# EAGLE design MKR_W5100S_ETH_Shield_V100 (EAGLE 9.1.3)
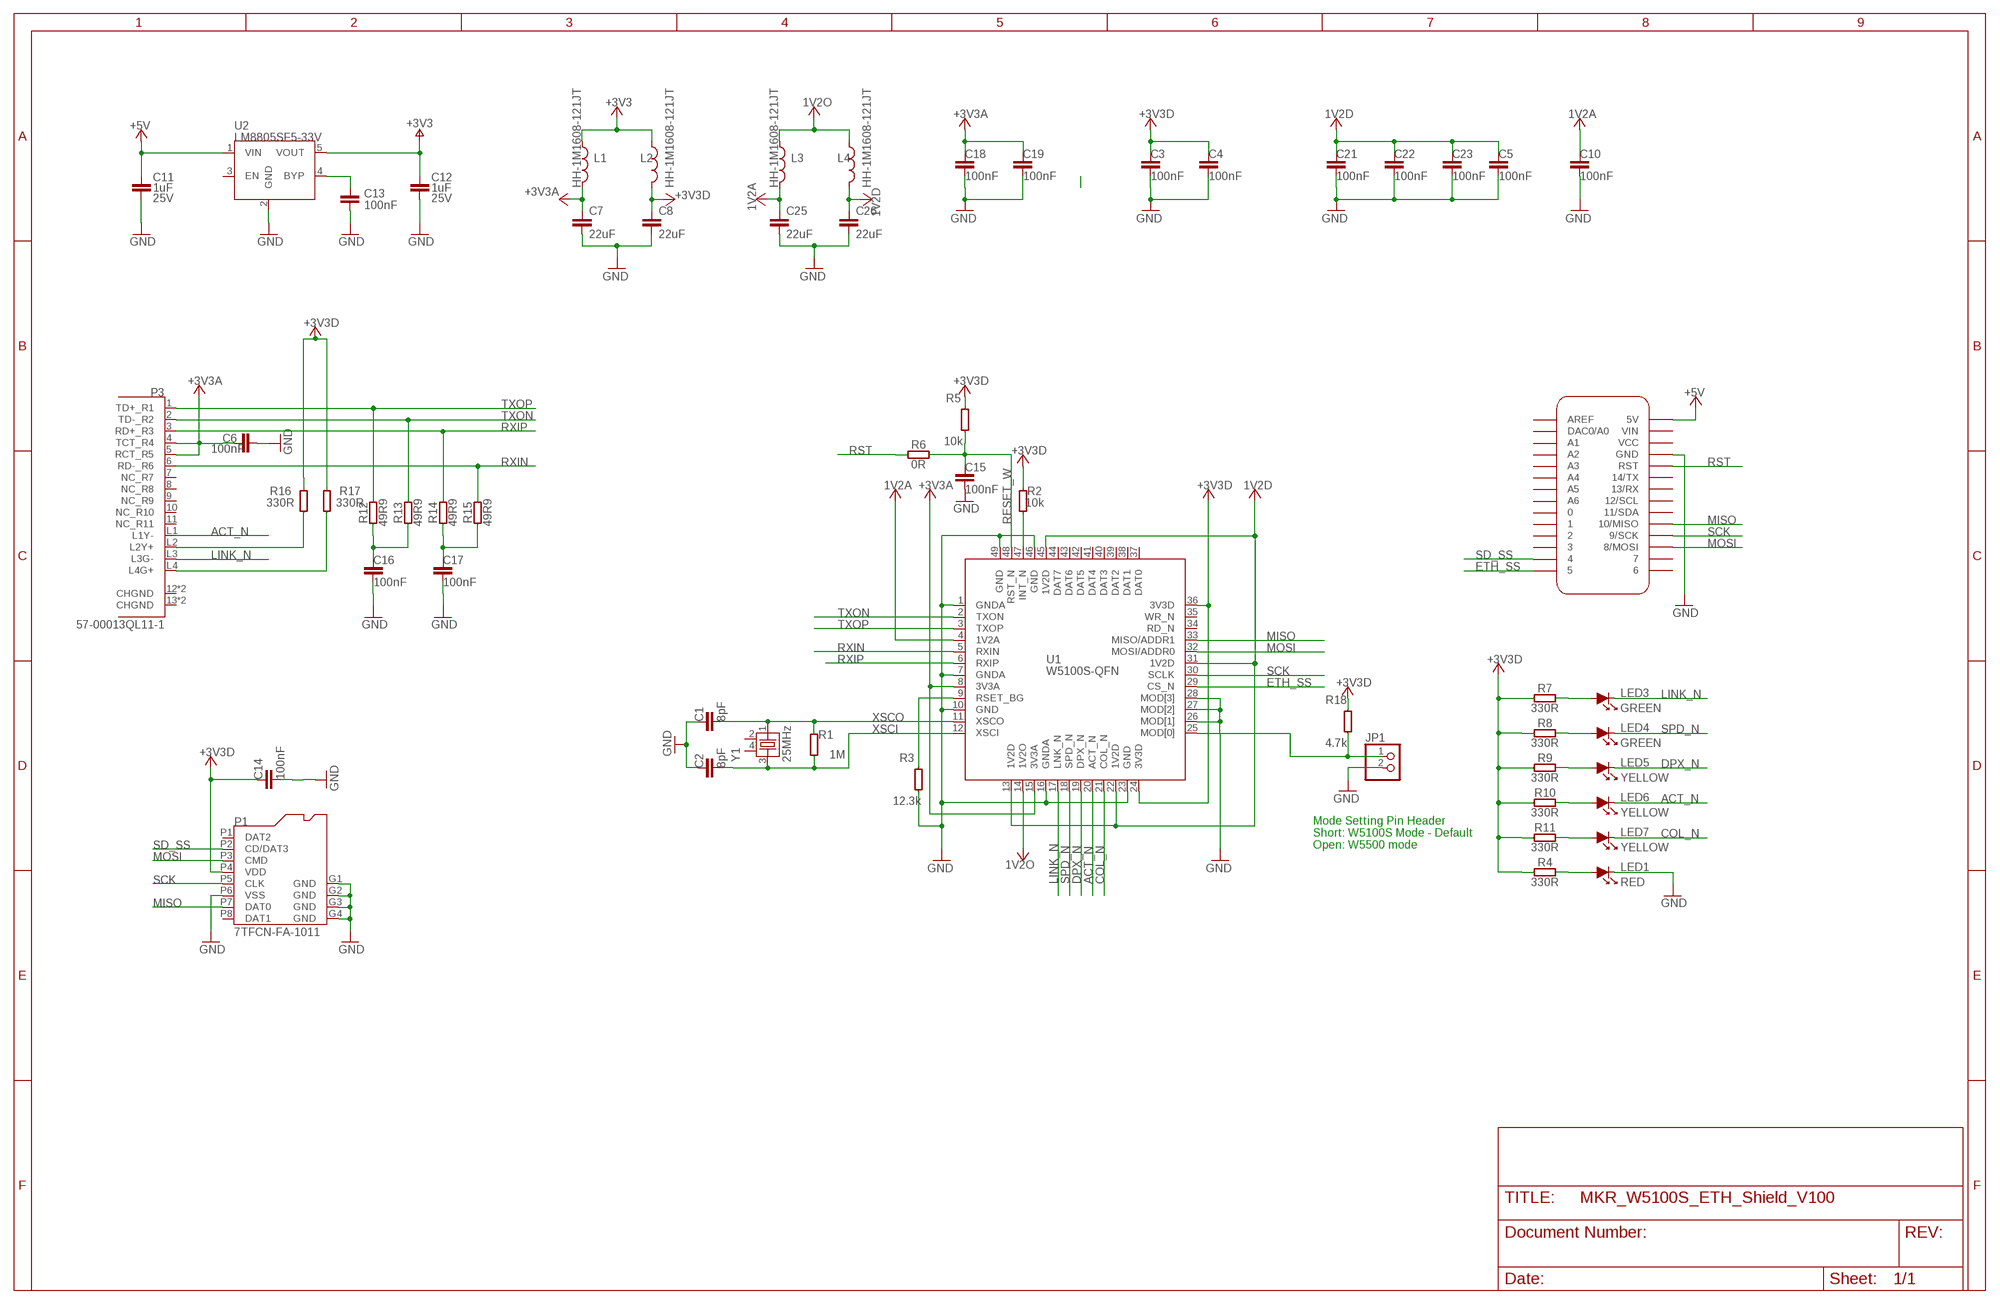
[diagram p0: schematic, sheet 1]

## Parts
C1  8pF  C-1UF-0402  [0402-1005X55N]
C2  8pF  C-1UF-0402  [0402-1005X55N]
C3  100nF  C-1UF-0402  [0402-1005X55N]
C4  100nF  C-1UF-0402  [0402-1005X55N]
C5  100nF  C-1UF-0402  [0402-1005X55N]
C6  100nF  C-1UF-0402  [0402-1005X55N]
C7  22uF  C-22U-0805  [0805-R2013X50N]
C8  22uF  C-22U-0805  [0805-R2013X50N]
C10  100nF  C-1UF-0402  [0402-1005X55N]
C11  1uF  C-1UF-0402  [0402-1005X55N]
C12  1uF  C-1UF-0402  [0402-1005X55N]
C13  100nF  C-100NF-0402  [0402-1005X55N]
C14  100nF  C-1UF-0402  [0402-1005X55N]
C15  100nF  C-1UF-0402  [0402-1005X55N]
C16  100nF  C-1UF-0402  [0402-1005X55N]
C17  100nF  C-1UF-0402  [0402-1005X55N]
C18  100nF  C-1UF-0402  [0402-1005X55N]
C19  100nF  C-1UF-0402  [0402-1005X55N]
C21  100nF  C-1UF-0402  [0402-1005X55N]
C22  100nF  C-1UF-0402  [0402-1005X55N]
C23  100nF  C-1UF-0402  [0402-1005X55N]
C25  22uF  C-22U-0805  [0805-R2013X50N]
C26  22uF  C-22U-0805  [0805-R2013X50N]
JP1  PINHD-1X2  [1X02]
L1  HH-1M1608-121JT  BLM18PG471SN1D  [0603-1608X90N]
L2  HH-1M1608-121JT  BLM18PG471SN1D  [0603-1608X90N]
L3  HH-1M1608-121JT  BLM18PG471SN1D  [0603-1608X90N]
L4  HH-1M1608-121JT  BLM18PG471SN1D  [0603-1608X90N]
LED1  RED  LED-1608  [LED-1608]
LED3  GREEN  LED-1608  [LED-1608]
LED4  GREEN  LED-1608  [LED-1608]
LED5  YELLOW  LED-1608  [LED-1608]
LED6  YELLOW  LED-1608  [LED-1608]
LED7  YELLOW  LED-1608  [LED-1608]
MKR1  DNP  ARDUINO-UTILITY_MKRBOARDNO-OUTLINE  [ARDUINO-UTILITY_MKRBOARD-NOOUTLINE]
P1  7TFCN-FA-1011  [7TFCN-FA-1011]
P3  57-00013QL11-1  [57-00013QL11-1]
R1  1M  R-330R-0402  [0402-1005X55N]
R2  10k  R-330R-0402  [0402-1005X55N]
R3  12.3k  R-330R-0402  [0402-1005X55N]
R4  330R  R-330R-0402  [0402-1005X55N]
R5  10k  R-330R-0402  [0402-1005X55N]
R6  0R  R-330R-0402  [0402-1005X55N]
R7  330R  R-330R-0402  [0402-1005X55N]
R8  330R  R-330R-0402  [0402-1005X55N]
R9  330R  R-330R-0402  [0402-1005X55N]
R10  330R  R-330R-0402  [0402-1005X55N]
R11  330R  R-330R-0402  [0402-1005X55N]
R12  49R9  R-330R-0402  [0402-1005X55N]
R13  49R9  R-330R-0402  [0402-1005X55N]
R14  49R9  R-330R-0402  [0402-1005X55N]
R15  49R9  R-330R-0402  [0402-1005X55N]
R16  330R  R-330R-0402  [0402-1005X55N]
R17  330R  R-330R-0402  [0402-1005X55N]
R18  4.7k  R-330R-0402  [0402-1005X55N]
U1  W5100S-QFN  [W5100S-QFN]
U2  LM8805SF5-33V  [SOT23-5L]
Y1  25MHz  XTAL3225  [XTAL3225]

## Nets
1V2A: C10.1 C25.1 L3.2 U1.4(1V2A)
1V2D: C5.1 C21.1 C22.1 C23.1 C26.1 L4.2 U1.13(1V2D) U1.22(1V2D) U1.31(1V2D) U1.45(1V2D)
1V2O: L3.1 L4.1 U1.14(1V2O)
+3V3 [power]: C12.1 L1.1 L2.1 U2.5(VOUT)
+3V3A [power]: C6.1 C7.1 C18.1 C19.1 L1.2 P3.4(TCT_R4) P3.5(RCT_R5) U1.8(3V3A) U1.15(3V3A)
+3V3D: C3.1 C4.1 C8.1 C14.1 L2.2 P1.P4(VDD) R2.1 R4.2 R5.2 R7.2 R8.2 R9.2 R10.2 R11.2 R16.1 R17.1 R18.2 U1.24(3V3D) U1.36(3V3D)
+5V: C11.1 MKR1.5V U2.1(VIN)
ACT_N: LED6.K P3.L1(L1Y-) U1.20(ACT_N)
COL_N: LED7.K U1.21(COL_N)
DPX_N: LED5.K U1.19(DPX_N)
ETH_SS: MKR1.5 U1.29(CS_N)
GND [gnd]: C1.1 C2.1 C3.2 C4.2 C5.2 C6.2 C7.2 C8.2 C10.2 C11.2 C12.2 C13.2 C14.2 C15.2 C16.2 C17.2 C18.2 C19.2 C21.2 C22.2 C23.2 C25.2 C26.2 JP1.2 LED1.K MKR1.GND P1.G1(GND) P1.G2(GND) P1.G3(GND) P1.G4(GND) P1.P6(VSS) R3.1 U1.1(GNDA) U1.7(GNDA) U1.10(GND) U1.16(GNDA) U1.23(GND) U1.26(MOD[1]) U1.27(MOD[2]) U1.28(MOD[3]) U1.46(GND) U1.49(GND) U2.2(GND)
LINK_N: LED3.K P3.L3(L3G-) U1.17(LNK_N)
MISO: MKR1.10(10/MISO) P1.P7(DAT0) U1.33(MISO/ADDR1)
MOSI: MKR1.8(8/MOSI) P1.P3(CMD) U1.32(MOSI/ADDR0)
N$1: LED3.A R7.1
N$2: P3.L2(L2Y+) R16.2
N$3: LED1.A R4.1
N$4: LED4.A R8.1
N$5: LED5.A R9.1
N$6: LED6.A R10.1
N$7: LED7.A R11.1
N$8: P3.L4(L4G+) R17.2
N$9: JP1.1 R18.1 U1.25(MOD[0])
N$11: C13.1 U2.4(BYP)
N$12: C16.1 R12.2 R13.2
N$15: C17.1 R14.2 R15.2
N$16: R2.2 U1.47(INT_N)
N$20: R3.2 U1.9(RSET_BG)
RESET_W: C15.1 R5.1 R6.1 U1.48(RST_N)
RST: MKR1.RST R6.2
RXIN: P3.6(RD-_R6) R15.1 U1.5(RXIN)
RXIP: P3.3(RD+_R3) R14.1 U1.6(RXIP)
SCK: MKR1.9(9/SCK) P1.P5(CLK) U1.30(SCLK)
SD_SS: MKR1.4 P1.P2(CD/DAT3)
SPD_N: LED4.K U1.18(SPD_N)
TXON: P3.2(TD-_R2) R13.1 U1.2(TXON)
TXOP: P3.1(TD+_R1) R12.1 U1.3(TXOP)
XSCI: C2.2 R1.1 U1.12(XSCI) Y1.3
XSCO: C1.2 R1.2 U1.11(XSCO) Y1.1
Unconnected: MKR1.0 MKR1.1 MKR1.2 MKR1.3 MKR1.6 MKR1.7 MKR1.11(11/SDA) MKR1.12(12/SCL) MKR1.13(13/RX) MKR1.14(14/TX) MKR1.A0(DAC0/A0) MKR1.A1 MKR1.A2 MKR1.A3 MKR1.A4 MKR1.A5 MKR1.A6 MKR1.AREF MKR1.VCC MKR1.VIN P1.P1(DAT2) P1.P8(DAT1) P3.7(NC_R7) P3.8(NC_R8) P3.9(NC_R9) P3.10(NC_R10) P3.11(NC_R11) P3.12(CHGND) P3.13(CHGND) P3.P$3(CHGND) P3.P$4(CHGND) U1.34(RD_N) U1.35(WR_N) U1.37(DAT0) U1.38(DAT1) U1.39(DAT2) U1.40(DAT3) U1.41(DAT4) U1.42(DAT5) U1.43(DAT6) U1.44(DAT7) U2.3(EN) Y1.2 Y1.4

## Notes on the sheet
- Mode Setting Pin Header
  Short: W5100S Mode - Default
  Open: W5500 mode

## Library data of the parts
C1-C6 C10-C12 C14-C19 C21-C23 = MK1_Zero:C: Capacitor; DESCR: CAP CER 1UF 25V 10% X5R 0402; MF: Murata; MPN: GRM155R61E105KA12D; VOLTAGE: 25V
C7 C8 C25 C26 = Arduino-rcl:C: SMD Capacitor; CODE-ARDUINO: 2233; DATASHEET: https://media.digikey.com/pdf/Data%20Sheets/Samsung%20PDFs/CL21A226MQCLQNC_character.pdf; DISTRIBUTOR-LINK: https://www.digikey.com/product-detail/en/samsung-electro-mechanics-america-inc/CL21A226MQCLQNC/1276-2412-1-ND/3890498; DISTRIBUTOR-PN: 1276-2412-1-ND; MANUFACTURER: Samsung; MANUFACTURER-PN: CL21A226MQCLQNC; VALUE: 22u
C13 = MK1_Zero:C: Capacitor; DESCR: CAP CER 0.1UF 50V 10% X5R 0402; MF: TDK; MPN: C1005X5R1H104K050BB
JP1 = PinHeader:PINHD-1X2: PIN HEADER
L1-L4 = MK1_Zero:BLM18PG471SN1D: FERRITE CHIP 470 OHM 1000MA 0603
LED1 LED3-LED7 = DIODE:LED-1608
MKR1 = MKRETHShieldV2.0:ARDUINO-UTILITY_MKRBOARD: MKR board footprint; DATASHEET: DNP; DISTRIBUTOR-LINK: DNP; DISTRIBUTOR-PN: DNP; MANUFACTURER: DNP; MANUFACTURER-PN: DNP
P1 = Connector:7TFCN-FA-1011
P3 = WIZnet:57-00013QL11-1
R1-R18 = MK1_Zero:R: Resistor; DESCR: RES 330 OHM 1/16W 1% 0402 SMD; MF: Yageo; MPN: RC0402FR-07330RL
U1 = WIZnet:W5100S-QFN
U2 = RECULATOR:LM8805SF5-33V
Y1 = X-TAL:XTAL3225

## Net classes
1 power: width 0.254 mm, drill 0.3 mm, clearance 0.127 mm
2 gnd: width 0.254 mm, drill 0.3 mm, clearance 0.127 mm

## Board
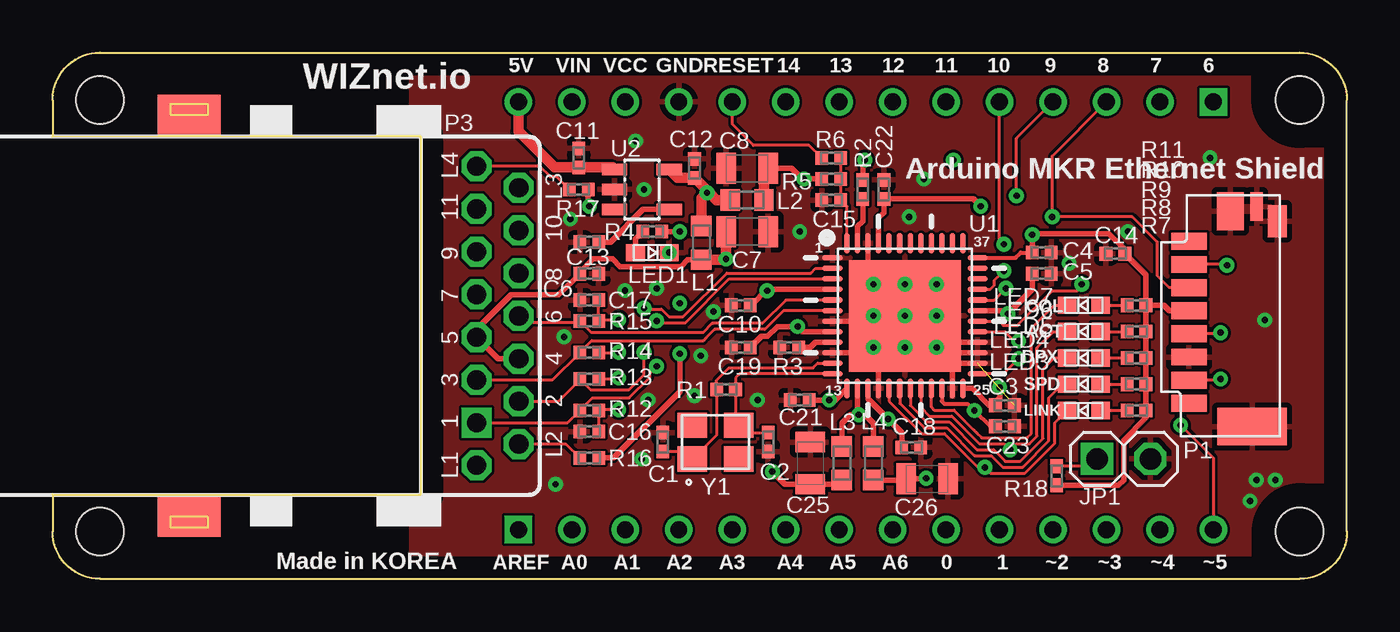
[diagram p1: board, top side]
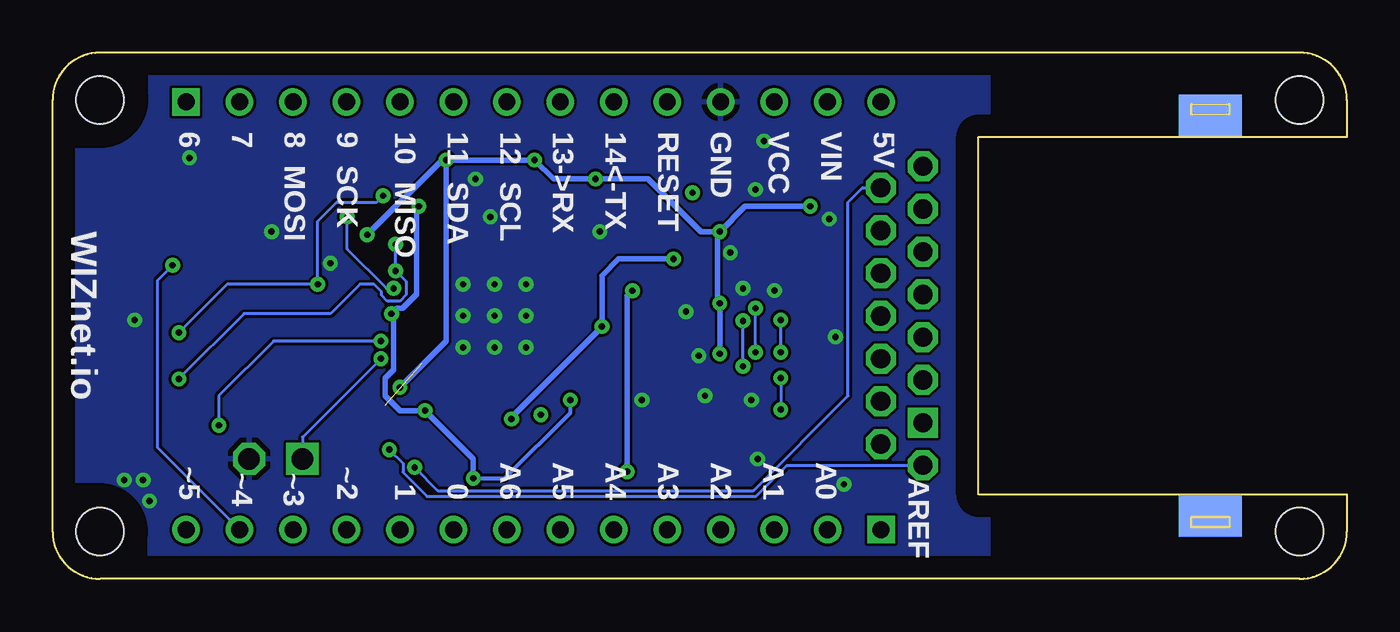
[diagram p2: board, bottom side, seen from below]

Size 61.5 x 25 mm. Coordinates in mm from the lower left corner, seen from the top.
Outline: 2.25,0 59.25,0 arc90 61.5,2.25 61.5,22.75 arc90 59.25,25 2.25,25 arc90 0,22.75 0,21 17.5,21 17.5,4 0,4 0,2.25 arc90 2.25,0
Copper layers (1*16): Top 0.035mm / dielectric 1.5mm / Bottom 0.035mm
Design rules "default *": minimum track width 6mil, minimum drill 0.3mm, track to track 5mil, track to pad 5mil, pad to pad 5mil, via to via 5mil, smd to smd 5mil, copper to edge 40mil, drill to drill 6mil, minimum pad ring 10mil, minimum via ring 8mil, stop-mask expansion 4mil, vias tented up to drill 15mil, thermal gap 10mil
Holes 2.25 mm at 2.25,2.25 2.25,22.75 59.25,2.25 59.25,22.75
tRestrict: area 57,20.5 to 61.5,25; area 57,0 to 61.5,4.5; 4 lines
bRestrict: area 57,20.5 to 61.5,25; area 57,0 to 61.5,4.5; 4 lines

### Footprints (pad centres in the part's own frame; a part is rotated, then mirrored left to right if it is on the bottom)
0402-1005X55N = smd 0.62 x 0.62: 1 -0.45,0; 2 0.45,0
0805-R2013X50N = smd 0.95 x 1.45: 1 -1,0; 2 1,0
1X02 = drill 1.016 square: 1 -1.27,0 | drill 1.016 octagon: 2 1.27,0
0603-1608X90N = smd 0.95 x 1: 1 -0.8,0; 2 0.8,0
LED-1608 = smd 0.89 x 0.82: A -0.8,0; K 0.8,0
ARDUINO-UTILITY_MKRBOARD-NOOUTLINE = drill 0.8: 0 42.455,2.34; 1 44.995,2.34; 2 47.535,2.34; 3 50.075,2.34; 4 52.615,2.34; 5 55.155,2.34; 5V 22.135,22.66; 7 52.615,22.66; 8 50.075,22.66; 9 47.535,22.66; 10 44.995,22.66; 11 42.455,22.66; 12 39.915,22.66; 13 37.375,22.66; 14 34.835,22.66; A0 24.675,2.34; A1 27.215,2.34; A2 29.755,2.34; A3 32.295,2.34; A4 34.835,2.34; A5 37.375,2.34; A6 39.915,2.34; GND 29.755,22.66; RST 32.295,22.66; VCC 27.215,22.66; VIN 24.675,22.66 | drill 0.8 square: 6 55.155,22.66; AREF 22.135,2.34
7TFCN-FA-1011 = smd 1.8 x 3.3: G1 -5.26,0 | smd 1.8 x 1.3: G2 4.97,1.04 | smd 1.36 x 0.6: G3 5.19,-0.21 | smd 1.5 x 0.9: G4 4.49,-1.2 | smd 0.8 x 1.7: P1 3.54,3; P2 2.44,3; P3 1.34,3; P4 0.24,3; P5 -0.86,3; P6 -1.96,3; P7 -3.06,3; P8 -4.16,3
57-00013QL11-1 = drill 0.914 square: 1 5.075,10.15 | drill 0.914 octagon: 2 4.065,12.15; 3 3.045,10.15; 4 2.035,12.15; 5 1.015,10.15; 6 0.005,12.15; 7 -1.015,10.15; 8 -2.025,12.15; 9 -3.045,10.15; 10 -4.055,12.15; 11 -5.075,10.15; L1 7.105,10.15; L2 6.095,12.15; L3 -6.085,12.15; L4 -7.105,10.15 | smd 2 x 3: 12 -9.5,-3.51; 13 9.5,-3.51 | smd 2 x 3 bottom: P$3 -9.5,-3.51; P$4 9.5,-3.51
W5100S-QFN = smd 0.95 x 0.25: 1 -3.45,2.75; 2 -3.45,2.25; 3 -3.45,1.75; 4 -3.45,1.25; 5 -3.45,0.75; 6 -3.45,0.25; 7 -3.45,-0.25; 8 -3.45,-0.75; 9 -3.45,-1.25; 10 -3.45,-1.75; 11 -3.45,-2.25; 12 -3.45,-2.75; 25 3.45,-2.75; 26 3.45,-2.25; 27 3.45,-1.75; 28 3.45,-1.25; 29 3.45,-0.75; 30 3.45,-0.25; 31 3.45,0.25; 32 3.45,0.75; 33 3.45,1.25; 34 3.45,1.75; 35 3.45,2.25; 36 3.45,2.75 | smd 0.25 x 0.95: 13 -2.75,-3.45; 14 -2.25,-3.45; 15 -1.75,-3.45; 16 -1.25,-3.45; 17 -0.75,-3.45; 18 -0.25,-3.45; 19 0.25,-3.45; 20 0.75,-3.45; 21 1.25,-3.45; 22 1.75,-3.45; 23 2.25,-3.45; 24 2.75,-3.45; 37 2.75,3.45; 38 2.25,3.45; 39 1.75,3.45; 40 1.25,3.45; 41 0.75,3.45; 42 0.25,3.45; 43 -0.25,3.45; 44 -0.75,3.45; 45 -1.25,3.45; 46 -1.75,3.45; 47 -2.25,3.45; 48 -2.75,3.45 | smd 5.3 x 5.3: 49 0,0
SOT23-5L = smd 0.55 x 1.2: 1 -0.95,-1.3; 2 0,-1.3; 3 0.95,-1.3; 4 0.95,1.3; 5 -0.95,1.3
XTAL3225 = smd 1.4 x 1.2: 1 -1.1,-0.8; 2 1.1,-0.8; 3 1.1,0.8; 4 -1.1,0.8

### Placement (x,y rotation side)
C1  29,6.5 270 top
C2  34,6.5 90 top
C3  45.25,8.25 0 top
C4  47,15.5 0 top
C5  47,14.5 0 top
C6  25.5,14.5 0 top
C7  33,16.5 0 top
C8  33,19.5 180 top
C10  32.7,13 180 top
C11  25,20 90 top
C12  30.5,19.5 90 top
C13  25.5,16 180 top
C14  50.5,15.45 180 top
C15  37,18 180 top
C16  25.5,7 180 top
C17  25.5,13.25 180 top
C18  40.8,6.25 0 top
C19  32.7,11 180 top
C21  35.5,8.5 180 top
C22  39.5,18.5 90 top
C23  45.25,7.25 0 top
C25  36,5.5 90 top
C26  41.55,4.75 0 top
JP1  50.9,5.7 0 top
L1  30.83,15.96 270 top
L2  33,18 0 top
L3  37.5,5.5 270 top
L4  39,5.5 270 top
LED1  28.5,15.5 0 top
LED3  49,8 180 top
LED4  49,9.25 180 top
LED5  49,10.5 180 top
LED6  49,11.75 180 top
LED7  49,13 180 top
MKR1  0,0 0 top
P1  57,12.5 90 top
P3  10,12.5 270 top
R1  32,9 180 top
R2  38.5,18.5 270 top
R3  35,11 0 top
R4  28.5,16.5 0 top
R5  37,19 180 top
R6  37,20 180 top
R7  51.5,8 0 top
R8  51.5,9.25 0 top
R9  51.5,10.5 0 top
R10  51.5,11.75 0 top
R11  51.5,13 0 top
R12  25.5,8 0 top
R13  25.5,9.5 0 top
R14  25.5,10.75 0 top
R15  25.5,12.25 0 top
R16  25.5,5.75 180 top
R17  25,18.5 180 top
R18  47.7,4.9 270 top
U1  40.5,12.5 0 top
U2  28,18.5 270 top
Y1  31.5,6.5 0 top

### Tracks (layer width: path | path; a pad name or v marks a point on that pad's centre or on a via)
1V2A  (via drill 0.3)
  Top 0.152: v33.95,13.69 33.95,13.75
  Top 0.254: U1.4 33.95,13.75 33.2,13 C10.1 | L3.2 37.3,4.5 C25.1 34.8,4.5 v34.2,5.1
  Bottom 0.254: v34.2,5.1 34.2,13.44 v33.95,13.69
1V2D  (via drill 0.3)
  Top 0.2: U1.22 42.25,8.45 42.38,8.32 43.48,8.32 v43.8,8 44.55,7.25 44.7,7.25 | 41.48,4.75 v41.51,4.78
  Top 0.254: U1.13 37.2,8.5 v36.9,8.5 C21.1 | 44.7,7.25 C23.1 | L4.2 40.5,4.7 C26.1 41.48,4.75 | U1.45 39.25,17.15 39.5,17.4 C22.1 43.75,18.05 v44.1,17.7 | U1.31 45.25,12.75 v45.4,12.6 46.55,13.75 C5.1
  Bottom 0.2: v41.51,4.78 40.02,4.78 36.9,7.9 v36.9,8.5
  Bottom 0.254: v41.51,4.78 41.51,5.71 v43.8,8 45,8 45.7,8.7 45.7,9.54 45.29,9.95 45.29,12.49 v45.4,12.6 45.13,12.87 44.86,12.87 44.2,13.53 44.2,17.6 v44.1,17.7
1V2O  (via drill 0.3)
  Top 0.254: U1.14 38.25,7.85 v38.3,7.8 | v38.3,7.8 37.9,7.8 37.5,7.4 L3.1 | v38.3,7.8 38.6,7.8 39,7.4 L4.1
+3V3  (via drill 0.3)
  Top 0.508: U2.5 29.7,19.05 C12.1 31.23,18.32 | 31.23,18.32 31.55,18 L2.1 | 31.23,18.32 | 31.23,18.32 31.11,18.32 v31.09,18.34 30.83,18.08 L1.1
+3V3A  (via drill 0.3)
  Top 0.254: U1.15 38.75,8.55 v39.7,7.6 40.35,6.95 C18.1 | U1.8 35.64,11.75 v35.4,11.99 34.44,11.99 33.98,11.53 33.68,11.53 C19.1 | L1.2 30.17,15.16 29.85,14.84 26.96,14.84 26.6,15.2 25.68,15.2 25.05,14.57 C6.1 24.05,13.5 21.79,13.5 20.15,11.86 P3.5 21.17,10.46 P3.4
  Top 0.508: L1.2 31.96,15.16 | 31.96,15.16 v32,15.2 | C7.1 v32,15.2 | v32,15.2 31.96,15.16
  Bottom 0.254: v32,15.2 34.6,15.2 35.4,14.4 v35.4,11.99 39.7,7.69 v39.7,7.6
+3V3D  (via drill 0.3)
  Top 0.152: v46.55,16.35 46.55,16.4
  Top 0.2: U1.36 45.75,15.25 46,15.5 C4.1
  Top 0.254: U1.24 43.7,9.05 44.5,8.25 C3.1 44.8,8.4 45,8.6 v45,9.1 | R11.2 R10.2 R9.2 R8.2 R7.2 51.95,7.65 50.9,6.6 50.9,4.7 50.65,4.45 R18.2 | P1.P4 53.06,12.74 52.8,13 R11.2 | R11.2 51.95,14.45 C14.1 50.95,15.65 50.2,16.4 46.55,16.4 C4.1 | R17.1 25.45,17.75 v25.5,17.7 | v29.8,16.5 R4.2 | C8.1 35.1,19.5 35.6,19 v35.7,19 R5.2 | v38.6,19.9 38.5,19.8 R2.1 | v29.8,10.7 29.8,8.9 26.65,5.75 R16.1 | v29.8,10.7 29.8,10.8 v29.8,10.7
  Top 0.508: L2.2 33.8,19.3 C8.1
  Bottom 0.254: v25.5,17.7 28.6,17.7 v29.8,16.5 29.9,16.5 29.91,16.5 | v35.7,19 35.9,19 | 35.9,19 37.7,19 v38.6,19.9 v42.8,19.9 | 29.91,16.5 30.7,16.5 33.2,19 35.9,19 | v42.8,19.9 43,19.9 v46.55,16.35 | v45,9.1 42.8,11.3 v42.8,19.9 | v29.8,10.7 v29.8,13.1 29.91,13.21 29.91,16.5
+5V
  Top 0.508: U2.1 26.6,19.55 C11.1 23.85,19.55 22.14,21.27 MKR1.5V
ACT_N  (via drill 0.3)
  Top 0.152: 41.25,8.69 U1.20 41.25,8.15 41.66,7.74 42.72,7.74 44.04,6.42 45.22,6.42 v45.5,6.14 45.78,6.42 46.42,6.42 46.78,6.78 46.78,10.98 47.55,11.75 LED6.K
  Bottom 0.152: v45.5,6.14 44.86,5.5 44.86,5.07 43.71,3.92 28.08,3.92 26.61,5.39 P3.L1
COL_N
  Top 0.152: U1.21 41.75,8.17 41.9,8.02 42.84,8.02 43.78,7.07 | 43.78,7.07 43.88,6.98 | 43.88,6.98 43.93,6.93 43.78,7.07 | 43.88,6.98 44.16,6.7 46.3,6.7 46.5,6.9 46.5,11.9 47.6,13 LED7.K
DPX_N
  Top 0.152: 40.75,8.69 U1.19 40.75,8.24 41.53,7.46 42.61,7.46 43.92,6.14 44.72,6.14 45.27,5.59 45.98,5.59 47.06,6.67 47.06,9.96 47.6,10.5 LED5.K
ETH_SS  (via drill 0.3)
  Top 0.152: U1.29 45.25,11.75 45.7,11.3 v45.9,11.3 | v53.6,7.3 55.16,5.75 MKR1.5
  Bottom 0.152: v45.9,11.3 51,11.3 53.6,8.7 v53.6,7.3
GND  (via drill 0.3)  (1 unrouted)
  Top 0.254: U1.28 42.25,11.25 42.1,11.1 | 42.1,11.1 v42,11 | U1.46 38.75,14.25 v39,14 | U1.10 38.75,10.75 v39,11 39.25,10.75 U1.16 | U1.7 38.75,12.25 v39,12.5 | U1.23 42.75,10.3 42.75,10.34 | 42.75,10.34 42.75,10.45 42.65,10.55 | 42.65,10.55 42.1,11.1 | U1.27 42.85,10.75 42.65,10.55 | U1.26 42.84,10.25 42.75,10.34
  other vias: 40.5,12.5 40.5,11 40.5,14 42,12.5 42,14 48.3,15 51.1,16.5 35.5,16.5 40.7,17.2 33.5,8.5 30.8,10.6 27.2,13.7 28.1,18.5 29.3,15.5 24.6,17.1 24.3,11.5 28.3,8.5 31.4,12.7 57.2,4.7 58.1,4.7 56.9,3.7 57.6,12.3 55,20 27.7,20.8 23.9,4.5 28,5.7 30.5,8.7 28.7,13.8 41.4,19
  pour Top: 17,-1 17,26 62,26 62,-1
  pour Bottom: 17,27 17,-2 63,-2 63,27
LINK_N  (via drill 0.3)
  Top 0.152: U1.17 39.75,8.45 41.3,6.9 42.38,6.9 43.98,5.3 v44.3,5.3 44.57,5.03 46.21,5.03 47.62,6.44 47.62,7.42 LED3.K
  Bottom 0.152: v44.3,5.3 43.2,4.2 28.2,4.2 23.7,8.7 23.7,17.9 23.02,18.59 P3.L3
MISO  (via drill 0.3)
  Top 0.152: v45.2,15.9 44.99,16.11 MKR1.10 | v55.5,9.5 55.44,9.44 P1.P7 | U1.33 44.55,13.75 44.74,13.94 44.74,14.18 v45.2,14.63
  Bottom 0.152: v55.5,9.5 52.4,12.6 48.3,12.6 46.9,14 46.23,14 45.88,13.65 45.88,13.48 45.6,13.2 45,13.2 44.7,13.5 44.7,14.13 v45.2,14.63 v45.2,15.9
MOSI  (via drill 0.3)
  Top 0.152: U1.32 44.75,13.25 v45.3,13.8 | MKR1.8 47.5,20.09 v47.5,17.2 51.3,17.2 52.5,16 52.5,14.4 53.06,13.84 P1.P3
  Bottom 0.152: v47.5,17.2 47.5,15.67 45.63,13.8 v45.3,13.8
N$1
  Top 0.152: R7.1 LED3.A
N$2
  Top 0.152: R16.2 24.39,6.41 P3.L2
N$3
  Top 0.254: R4.1 27.7,16.15 LED1.A
N$4
  Top 0.152: LED4.A R8.1
N$5
  Top 0.152: LED5.A R9.1
N$6
  Top 0.152: LED6.A R10.1
N$7
  Top 0.152: LED7.A R11.1
N$8
  Top 0.152: R17.2 23.96,19.09 23.66,19.09 23.15,19.61 P3.L4
N$9  (via drill 0.3)
  Top 0.152: JP1.1 49.28,5.35 R18.1 | 45.68,10.25 v45.9,10.47 45.18,9.75 U1.25
  Bottom 0.152: v45.9,10.47 49.63,6.74 JP1.1
N$11
  Top 0.254: U2.4 28.05,17.55 26.5,16 C13.1
N$12  (via drill 0.3)
  Top 0.152: R13.2 26.86,9.5 v26.9,9.54 | v26.9,8.04 25.99,8.04 R12.2 C16.1
  Bottom 0.152: v26.9,9.54 v26.9,8.04
N$15  (via drill 0.3)
  Top 0.152: R14.2 26.89,10.75 v26.9,10.76 | v26.9,12.3 26,12.3 R15.2 C17.1
  Bottom 0.152: v26.9,10.76 v26.9,12.3
N$16
  Top 0.254: U1.47 38.25,16.75 38.5,17 R2.2
N$20
  Top 0.254: U1.9 36.25,11.25 36,11 R3.2
RESET_W
  Top 0.152: U1.48 37.75,17.7 C15.1 R5.1 R6.1
RST
  Top 0.152: R6.2 35.95,20.6 33.3,20.6 32.3,21.61 MKR1.RST
RXIN
  Top 0.152: U1.5 34.84,13.25 33.73,12.14 31.4,12.14 | 31.4,12.14 31.34,12.14 | 31.34,12.14 | 31.4,12.14 31.34,12.14 | 31.34,12.14 30.91,11.7 25.6,11.7 25.44,11.86 25.1,12.2 | 25.1,12.2 R15.1 | P3.6 22.45,12.2 25.1,12.2
RXIP
  Top 0.152: U1.6 34.73,12.75 33.84,11.86 31.46,11.86 31.05,11.45 30.92,11.32 25.62,11.32 25.44,11.14 R14.1 23.75,9.46 P3.3
SCK  (via drill 0.3)
  Top 0.152: v55.5,11.7 55.44,11.64 P1.P5 | v45.8,18.2 45.8,20.93 MKR1.9 | v48.9,14 48.9,13.9 48.7,13.7 47.5,13.7 45.84,12.04 45.17,12.04 44.96,12.25 U1.30
  Bottom 0.152: v55.5,11.7 53.2,14 v48.9,14 48.9,17 48,17.9 46.1,17.9 v45.8,18.2
SD_SS  (via drill 0.3)
  Top 0.152: v55.8,14.9 55.76,14.94 P1.P2
  Bottom 0.152: MKR1.4 56.5,6.22 56.5,14.2 v55.8,14.9
SPD_N
  Top 0.152: 40.25,8.7 U1.18 40.25,8.35 41.42,7.18 42.49,7.18 43.81,5.86 44.6,5.86 45.15,5.31 46.09,5.31 47.34,6.55 47.34,8.6 47.99,9.25 LED4.K
TXON  (via drill 0.3)
  Top 0.152: R13.1 25.07,9.47 | 25.07,9.47 25.44,9.11 25.56,8.99 27.39,8.99 28.1,9.7 v28.1,10.76 | v28.1,12.86 28.14,12.81 28.93,12.81 29.3,12.45 29.95,12.45 32.03,14.53 36.03,14.53 36.25,14.75 U1.2 | P3.2 24.04,8.44 25.07,9.47
  Bottom 0.152: v28.1,10.76 v28.1,12.86
TXOP  (via drill 0.3)
  Top 0.152: U1.3 32.15,14.25 30.07,12.17 28.79,12.17 v28.7,12.26 | v28.7,10.1 28.38,9.78 28.38,9.58 27.39,8.6 25.65,8.6 25.44,8.39 R12.1 24.48,7.42 P3.1
  Bottom 0.152: v28.7,10.1 v28.7,12.26
XSCI
  Top 0.152: U1.12 32.65,9.75 32.45,9.55 R1.1 32.45,7.45 Y1.3 32.95,6.95 C2.2
XSCO
  Top 0.152: C1.2 30.05,6.05 Y1.1 30.42,5.7 31.55,6.83 R1.2 31.55,9.45 32.13,10.03 36.13,10.03 36.35,10.25 U1.11

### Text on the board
tNames: Y1
tsilk: 5V | VIN | VCC | GND | RESET | 14 | 13 | 12 | 11 | 10 | 9 | 8 | 7 | 6 | WIZnet.io | Arduino MKR Ethernet Shield | COL | ACT | DPX | SPD | LINK | Made in KOREA | AREF | A0 | A1 | A2 | A3 | A4 | A5 | A6 | 0 | 1 | ~2 | ~3 | ~4 | ~5
bsilk: 5V | VIN | VCC | GND | RESET | 14<-TX | 13->RX | 12 SCL | 11 SDA | 10 MISO | 9 SCK | 8 MOSI | 7 | 6 | WIZnet.io | A0 | A1 | A2 | A3 | A4 | A5 | A6 | 0 | 1 | ~2 | ~5 | ~3 | ~4 | AREF

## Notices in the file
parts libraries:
Arduino-rcl: Copyright (c) 2016-2017 Arduino LLC. All right reserved.
